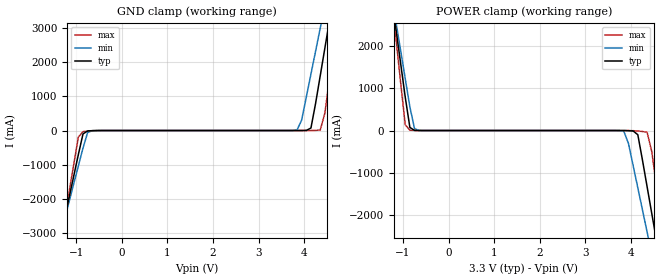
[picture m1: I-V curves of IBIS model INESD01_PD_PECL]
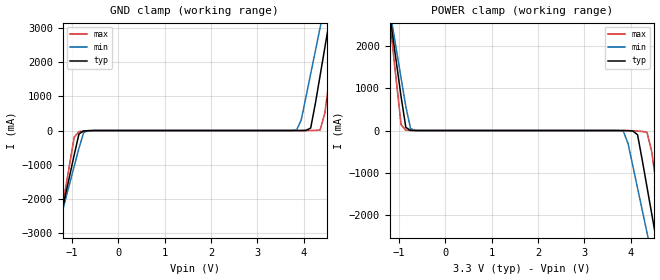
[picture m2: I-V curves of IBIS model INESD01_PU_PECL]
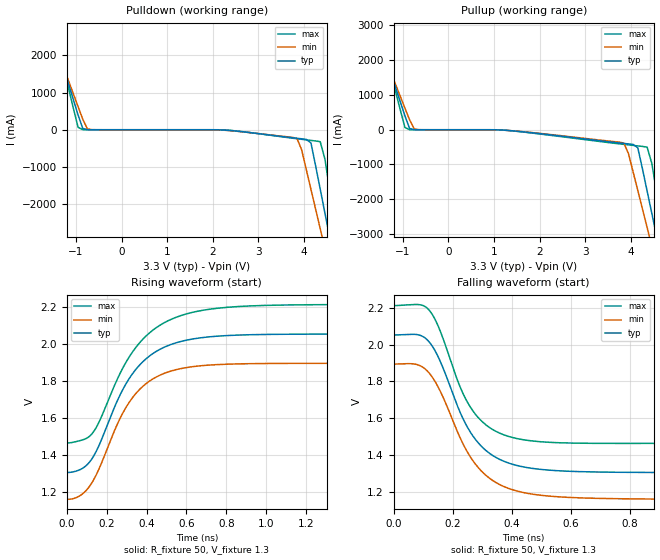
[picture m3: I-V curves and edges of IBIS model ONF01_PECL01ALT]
|   This file is an IBIS representation of the   |
|   Integrated Devices Technology, Inc.   |
|   ICS85357I-01   |
|   4:1 OR 2:1 DIFFERENTIAL-TO-3.3V LVPECL / ECL CLOCK MULTIPLEXER   |
[IBIS Ver]   4.1
[File name]   85357i_01_3v3.ibs
[File Rev]   1.0
[Date]   5 Jan 2009 | Last modified
|   18 Jan 2002 | Generated
[Source]   Originated at Integrated Devices Technology, Inc.
[Disclaimer]
IDT hereby grants the user of this IBIS model a non-exclusive,
nontransferable license to use this IBIS model under the following terms.
Before using this IBIS model, the user should read this license.
If the user does not accept these terms,  the IBIS model should be
returned to IDT within 30 days.
   The user is granted this license only to use the IBIS model and
is not granted rights to sell, load, rent, lease or license the IBIS
model in whole or in part, or in modified form to anyone other than
user. User may modify the IBIS model to suit its specific
applications but rights to derivative works and such modifications
shall belong to IDT.
   This IBIS model is provided on an "AS IS" basis and IDT makes
absolutely no warranty with respect to the information contained
herein. IDT DISCLAIMS AND CUSTOMER WAIVES ALL WARRANTIES, EXPRESS
OR IMPLIED, INCLUDING WARRANTIES OF MERCHANTABILITY OR FITNESS FOR
A PARTICULAR PURPOSE. The entire risk as to quality and performance
is with the Customer. ACCORDINGLY, IN NO EVENT SHALL THE COMPANY BE
LIABLE FOR ANY DAMAGES, WHETHER IN CONTRACT OR TORT,INCLUDING ANY
LOST PROFITS OR OTHER INCIDENTAL, CONSEQUENTIAL, EXEMPLARY, OR
PUNITIVE DAMAGES ARISING OUT OF THE USE OR APPLICATION OF THE IBIS
model provided in this package. Further, IDT reserves the right to
make changes without notice to any product herein to improve
reliability, function, or design. IDT does not convey any license
under patent rights or any other intellectual property rights,
including those of third parties.
   IDT is not obligated to provide maintenance or support
for the licensed IBIS model.
[Copyright]   Copyright 2002 by Integrated Devices Technology, Inc.
[Component]   ICS85357IG-01
[Manufacturer] Integrated Devices Technology, Inc.
[Package]
|TSSOP 20 Lead
|   typ   min   max
R_pkg   51.85m   41.1m   62.6m
L_pkg   1.568nH   0.734nH   2.401nH
C_pkg   0.221pF   0.068pF   0.373pF
[Pin]   signal_name   model_name   R_pin   L_pin   C_pin
1   VCC   POWER   62.6m   2.401n   0.373p
2   CLK0   INESD01_PD_PECL   57.23m   1.985n   0.297p
3   nCLK0   INESD01_PU_PECL   51.85m   1.568n   0.221p
4   CLK1   INESD01_PD_PECL   46.78m   1.151n   0.145p
5   nCLK1   INESD01_PU_PECL   41.1m   0.734n   0.068p
6   CLK2   INESD01_PD_PECL   41.1m   0.734n   0.068p
7   nCLK2   INESD01_PU_PECL   46.78m   1.151n   0.145p
8   CLK3   INESD01_PD_PECL   51.85m   1.568n   0.221p
9   nCLK3   INESD01_PU_PECL   57.23m   1.985n   0.297p
10   VEE   GND   62.6m   2.401n   0.373p
11   VEE   GND   62.6m   2.401n   0.373p
12   nc   nc   57.23m   1.985n   0.297p
13   nc   nc   51.85m   1.568n   0.221p
14   VCC   POWER   46.78m   1.151n   0.145p
15   nQ0   ONF01_PECL01ALT   41.1m   0.734n   0.068p
16   Q0   ONF01_PECL01ALT   41.1m   0.734n   0.068p
17   VCC   POWER   46.78m   1.151n   0.145p
18   SEL0   INESD01_PD_PECL   51.85m   1.568n   0.221p
19   SEL1   INESD01_PD_PECL   57.23m   1.985n   0.297p
20   VCC   POWER   62.6m   2.401n   0.373p
[Diff Pin]  inv_pin  vdiff tdelay_typ tdelay_min  tdelay_max
16   15   NA   0  0  0
2   3   0.15  0  0  0
4   5   0.15  0  0  0
6   7   0.6  0  0  0
8   9   0.6  0  0  0
| Models and submodels in the file (3): INESD01_PD_PECL (Input), INESD01_PU_PECL (Input), ONF01_PECL01ALT (Output_ECL)
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[Model]   INESD01_PD_PECL
Model_type  Input
Polarity   Non-Inverting
Vinl = 0.8V
Vinh = 2.0V
|   typ   min   max
C_comp   2pF   1.5pF   2.5pF
|   typ   min   max
[Voltage range]  3.3V   3.15V   3.45V
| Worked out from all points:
|   GND clamp passes 1 mA (typ) near -0.55 V on its own axis
|   POWER clamp passes 1 mA (typ) near -0.66 V on its own axis
[GND_clamp]
|Voltage   I(typ)   I(min)   I(max)
-2.586V   -10.86A    -9.487A    -13.15A
-1.361V   -3.24A     -3.145A    -3.432A
-1.259V   -2.606A    -2.617A    -2.622A
-952.6mV  -705.3mA   -1.038A    -192.4mA
-850.5mV  -99.9mA    -513.5mA   -31.23mA
-646.4mV  -3.788mA   -3.549mA   -8.297mA
3.844V    129.1uA    13.13mA    71.12uA
4.151V    73.33mA    1.652A     864.7uA
4.355V    1.607A     3.003A     15.44mA
4.559V    3.233A     4.356A     1.553A
4.763V    4.861A     5.711A     3.635A
5.375V    9.757A     9.783A     9.893A
[POWER_clamp]
|Voltage   I(typ)   I(min)   I(max)
-2.177V   10.57A     9.364A     12.62A
-1.157V   2.42A      2.586A     2.194A
-952.6mV  795.8mA    1.237A     137.8mA
-850.5mV  73.33mA    563.2mA    8.145mA
-646.4mV  535.8uA    2.004mA    431.2uA
3.844V    -826.3uA   -18.14mA   -47.07uA
4.151V    -99.9mA    -1.362A    -11.82mA
4.355V    -1.338A    -2.415A    -41.71mA
4.559V    -2.606A    -3.47A     -1.312A
4.661V    -3.24A     -3.998A    -2.123A
4.763V    -3.875A    -4.526A    -2.933A
5.579V    -8.954A    -8.756A    -9.414A
[Model]   INESD01_PU_PECL
Model_type  Input
Polarity   Non-Inverting
Vinl = 0.8V
Vinh = 2.0V
|   typ   min   max
C_comp   2pF   1.5pF   2.5pF
|   typ   min   max
[Voltage range]  3.3V   3.15V   3.45V
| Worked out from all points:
|   GND clamp passes 1 mA (typ) near -0.55 V on its own axis
|   POWER clamp passes 1 mA (typ) near -0.67 V on its own axis
[GND_clamp]
|Voltage   I(typ)   I(min)   I(max)
-3.3V     -15.3A     -13.19A    -18.82A
-1.361V   -3.24A     -3.145A    -3.432A
-1.259V   -2.606A    -2.617A    -2.622A
-952.6mV  -705.4mA   -1.038A    -192.5mA
-850.5mV  -99.96mA   -513.6mA   -31.29mA
-646.4mV  -3.852mA   -3.611mA   -8.361mA
3.844V    64.83uA    13.07mA    7.183uA
4.151V    73.26mA    1.652A     800.8uA
4.355V    1.607A     3.003A     15.37mA
4.559V    3.233A     4.356A     1.553A
4.763V    4.861A     5.711A     3.635A
6.6V      19.56A     17.94A     22.42A
[POWER_clamp]
|Voltage   I(typ)   I(min)   I(max)
-3.3V     19.56A     16.84A     24.11A
-1.259V   3.233A     3.262A     3.235A
-1.157V   2.419A     2.586A     2.194A
-952.6mV  795.8mA    1.236A     137.7mA
-850.5mV  73.26mA    563.1mA    8.081mA
-646.4mV  471.5uA    1.942mA    367.2uA
3.844V    -890.5uA   -18.21mA   -111uA
4.151V    -99.96mA   -1.362A    -11.88mA
4.355V    -1.338A    -2.415A    -41.77mA
4.559V    -2.606A    -3.47A     -1.313A
4.763V    -3.875A    -4.526A    -2.933A
6.6V      -15.3A     -14.05A    -17.51A
[Model]   ONF01_PECL01ALT
Model_type  Output_ECL
Polarity   Non-Inverting
Vmeas = 1.636
Rref = 50
Cref = 0
Vref = 1.3
|Variable  typ   min   max
C_comp   2p   1.5p   2.5p
[Voltage Range]   3.3   3.135   3.465
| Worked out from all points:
|   rising waveform, R_fixture 50, V_fixture 1.3: 20-80 % time 218ps typ, 206ps min, 242ps max; typ from 1.31 V to 2.05 V
|   falling waveform, R_fixture 50, V_fixture 1.3: 20-80 % time 134ps typ, 143ps min, 120ps max; typ from 2.05 V to 1.31 V
| Open source, no load
|  Voltage   I(typ)   I(min)   I(max)
[Pullup]
-3.3V     9.786A     8.45A      12.03A
-1.667V   3.247A     2.997A     3.691A
-1.565V   2.839A     2.657A     3.17A
-952.6mV  398mA      622.1mA    64.71mA
-850.5mV  36.63mA    284.2mA    1.532mA
-646.4mV  229.3uA    1.611mA    19.07uA
3.844V    -394.4mA   -383.6mA   -421.3mA
4.151V    -517.8mA   -1.749A    -465.4mA
4.355V    -1.764A    -2.812A    -500.3mA
4.559V    -3.036A    -3.875A    -1.773A
4.763V    -4.308A    -4.937A    -3.393A
6.6V      -15.79A    -14.52A    -18.03A
[Pulldown]
-3.3V     9.786A     8.45A      12.03A
-1.565V   2.839A     2.657A     3.17A
-1.463V   2.432A     2.317A     2.65A
-952.6mV  398mA      622.1mA    64.71mA
-850.5mV  36.63mA    284.2mA    1.532mA
-646.4mV  229.3uA    1.611mA    19.07uA
3.844V    -229.1mA   -232.1mA   -241.8mA
4.151V    -352.7mA   -1.598A    -286.7mA
4.355V    -1.599A    -2.66A     -322.1mA
4.559V    -2.871A    -3.722A    -1.595A
4.763V    -4.144A    -4.785A    -3.217A
6.6V      -15.69A    -14.41A    -17.97A
[Ramp]
|   typ   min   max
dV/dt_r   0.45V/0.37ns   0.45V/0.405ns   0.45V/0.27ns
dV/dt_f   0.45V/0.37ns   0.45V/0.405ns   0.45V/0.27ns
R_load =   50.0000
[Rising Waveform]
R_fixture = 50
V_fixture = 1.3   | VCC_typ - 2V
V_fixture_max = 1.465   | VCC_max - 2V
V_fixture_min = 1.135   | VCC_min - 2V
C_fixture = 0.0p
| Time   typ   min   max
0s        1.306V     1.161V     1.465V
70ps      1.323V     1.183V     1.479V
128ps     1.383V     1.254V     1.517V
258ps     1.703V     1.577V     1.819V
316ps     1.817V     1.689V     1.934V
398ps     1.919V     1.785V     2.042V
504ps     1.988V     1.846V     2.121V
658ps     2.03V      1.879V     2.175V
875ps     2.047V     1.891V     2.201V
2ns       2.052V     1.894V     2.211V
[Falling Waveform]
R_fixture = 50
V_fixture = 1.3   | VCC_typ - 2V
V_fixture_max = 1.465   | VCC_max - 2V
V_fixture_min = 1.135   | VCC_min - 2V
C_fixture = 0.0p
0s        2.052V     1.894V     2.211V
76ps      2.055V     1.893V     2.217V
118ps     2.018V     1.85V      2.19V
150ps     1.936V     1.772V     2.103V
222ps     1.644V     1.505V     1.782V
264ps     1.514V     1.38V      1.65V
326ps     1.409V     1.274V     1.549V
410ps     1.348V     1.21V      1.493V
708ps     1.309V     1.166V     1.465V
2ns       1.306V     1.161V     1.465V
